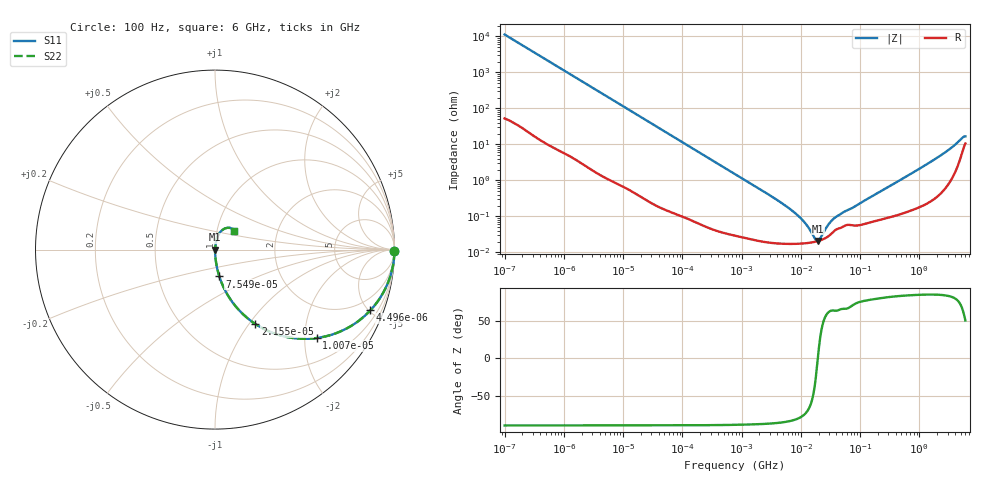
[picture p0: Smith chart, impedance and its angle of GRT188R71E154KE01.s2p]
!Murata Part Number: GRT188R71E154KE01
!These Parameters are Measured in Series Mode Connection
!Data Generated on Jun 19, 2026
!  o--ll--o
!Port1  Port2
!  o------o
!Operation Temp=25[degC], DC Bias Voltage=0[V]
!Freq. Start=100[Hz] Stop=6[GHz] 401[Steps]
# Hz S RI R 50
!Freq.(Hz) S11(Real) S11(Imag) S21(Real) S21(Imag) S12(Real) S12(Imag) S22(Real) S22(Imag)
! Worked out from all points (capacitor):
!   401 points, 100 Hz to 6 GHz, reference 50 ohm
!   read as one part in series: C = 140 nF near 109 Hz
!   lowest |Z| = 20.7 mohm at 19.46 MHz (marker M1)
!   series resonance near 19.37 MHz, so ESL is about 480 pH
!   S11 on the Smith chart (normalised r, x): 100 Hz: open; 4.496 kHz: 1.03, -5.11; 10.07 kHz: 1.01, -2.29; 21.55 kHz: 1.01, -1.07; 75.5 kHz: 1.00, -0.31; 6 GHz: 1.21, +0.26
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100  0.9999 -0.00882  0.000119 0.00882  0.000119 0.00882  0.9999 -0.00882
600  0.997 -0.0524  0.003 0.0524  0.003 0.0524  0.997 -0.0524
2008  0.9693 -0.1698  0.0307 0.1698  0.0307 0.1698  0.9693 -0.1698
4496  0.8657 -0.3384  0.1343 0.3384  0.1343 0.3384  0.8657 -0.3384
10066  0.5662 -0.4927  0.4338 0.4927  0.4338 0.4927  0.5662 -0.4927
21550  0.2244 -0.4142  0.7756 0.4142  0.7756 0.4142  0.2244 -0.4142
40335  0.0774 -0.2641  0.9226 0.2641  0.9226 0.2641  0.0774 -0.2641
75495  0.0241 -0.1497  0.9759 0.1497  0.9759 0.1497  0.0241 -0.1497
202169  0.0039 -0.0574  0.9961 0.0574  0.9961 0.0574  0.0039 -0.0574
774597  0.000519 -0.0151  0.9995 0.0151  0.9995 0.0151  0.000519 -0.0151
6948629  0.000174 -0.00149  0.9998 0.00149  0.9998 0.00149  0.000174 -0.00149
1.137099e7  0.000178 -0.000684  0.9998 0.000684  0.9998 0.000684  0.000178 -0.000684
1.555665e7  0.00019 -0.000271  0.9998 0.000271  0.9998 0.000271  0.00019 -0.000271
1.779312e7  0.000199 -0.000104  0.9998 0.000104  0.9998 0.000104  0.000199 -0.000104
1.946e7  0.000206 6e-06  0.9998 -6e-06  0.9998 -6e-06  0.000206 6e-06
2.128304e7  0.000216 0.000116  0.9998 -0.000116  0.9998 -0.000116  0.000216 0.000116
3.045065e7  0.000296 0.000576  0.9997 -0.000576  0.9997 -0.000576  0.000296 0.000576
3.80911e7  0.000415 0.000841  0.9996 -0.000841  0.9996 -0.000841  0.000415 0.000841
3.124326e8  0.000981 0.00677  0.999 -0.00677  0.999 -0.00677  0.000981 0.00677
3.205649e9  0.0135 0.0707  0.9865 -0.0707  0.9865 -0.0707  0.0135 0.0707
5.245841e9  0.0691 0.1215  0.9309 -0.1215  0.9309 -0.1215  0.0691 0.1215
6e9  0.1082 0.1046  0.8918 -0.1046  0.8918 -0.1046  0.1082 0.1046
